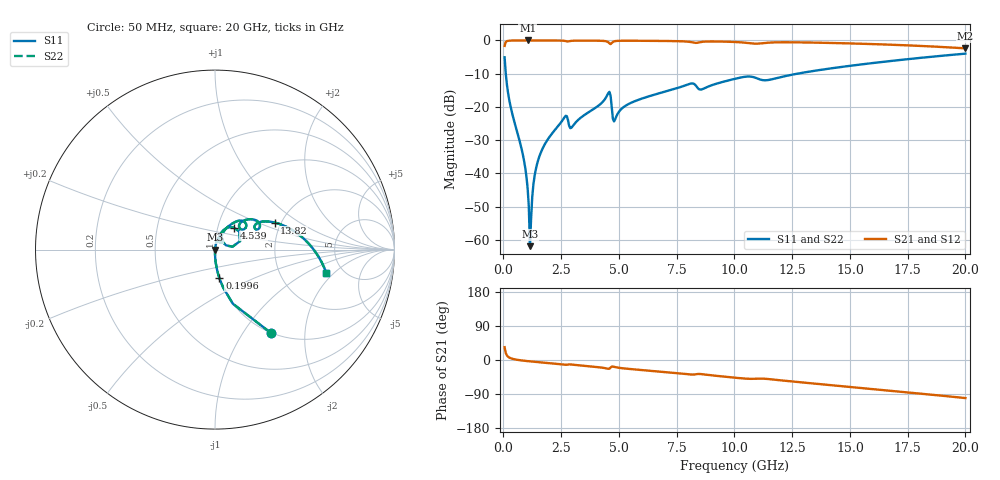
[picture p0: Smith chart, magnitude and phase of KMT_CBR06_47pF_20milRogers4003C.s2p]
! Data measured by Modelithics Inc. support@modelithics.com 813-866-6335
! KEMET CBR0603 47pF, Pad Width= 0.851mm, Pad Length= 0.64mm, Pad Gap= 0.62mm, 20mil Rogers 4003C substrate Data, January 2022
# hz S ma R 50
! 2 Port Network Data from SP1.SP block
! freq  magS11  angS11  magS21  angS21  magS12  angS12  magS22  angS22
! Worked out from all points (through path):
!   401 points, 50 MHz to 20 GHz, reference 50 ohm
!   highest |S21| = -0.01 dB at 1.048 GHz (marker M1); lowest = -2.4 dB at 20 GHz (marker M2)
!   group delay of S21, straight-line fit = 14 ps
!   lowest |S11| = -61.9 dB at 1.147 GHz (marker M3), VSWR 1.00, Z = 50.1 - j0.0562 ohm
!   |S11| at or under -10 dB: 100.6 MHz to 12.73 GHz (12.63 GHz wide, 197 % of centre)
!   |S22| runs from -61.9 to -4.0 dB; largest |S21 - S12| = 0
!   S11 on the Smith chart (normalised r, x): 50 MHz: 1.00, -1.34; 199.6 MHz: 1.00, -0.33; 4.539 GHz: 1.19, +0.30; 13.82 GHz: 1.85, +0.64; 20 GHz: 3.72, -1.60
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5e7  0.5586 -56.2  0.8291 33.8  0.8291 33.8  0.5586 -56.2
1.99625e8  0.1619 -81.2  0.9865 8.7  0.9865 8.7  0.1619 -81.2
8.48e8  0.01857 -90.0  0.9993 -1.6  0.9993 -1.6  0.01857 -90.0
9.97625e8  0.008804 -89.0  0.9994 -2.7  0.9994 -2.7  0.008804 -89.0
1.0475e9  0.005925 -87.4  0.9994 -3.0  0.9994 -3.0  0.005925 -87.4
1.14725e9  0.0008034 -44.3  0.9993 -3.6  0.9993 -3.6  0.0008034 -44.3
1.247e9  0.00447 77.6  0.9993 -4.2  0.9993 -4.2  0.00447 77.6
1.34675e9  0.009075 81.0  0.9992 -4.8  0.9992 -4.8  0.009075 81.0
1.4465e9  0.01345 81.7  0.9992 -5.4  0.9992 -5.4  0.01345 81.7
1.795625e9  0.02763 81.0  0.9987 -7.3  0.9987 -7.3  0.02763 81.0
2.6435e9  0.06992 67.9  0.9857 -12.3  0.9857 -12.3  0.06992 67.9
2.94275e9  0.0486 63.0  0.9862 -12.0  0.9862 -12.0  0.0486 63.0
3.391625e9  0.07074 72.8  0.9943 -14.8  0.9943 -14.8  0.07074 72.8
4.53875e9  0.1612 49.6  0.9401 -23.2  0.9401 -23.2  0.1612 49.6
4.838e9  0.06542 52.4  0.9768 -18.8  0.9768 -18.8  0.06542 52.4
5.386625e9  0.1091 64.7  0.99 -23.2  0.99 -23.2  0.1091 64.7
6.73325e9  0.16 58.5  0.9839 -30.4  0.9839 -30.4  0.16 58.5
1.0025e10  0.2648 39.8  0.9477 -46.7  0.9477 -46.7  0.2648 39.8
1.336662e10  0.345 26.8  0.9289 -61.7  0.9289 -61.7  0.345 26.8
1.38155e10  0.3644 24.5  0.9224 -64.2  0.9224 -64.2  0.3644 24.5
1.670825e10  0.4882 8.4  0.8643 -80.7  0.8643 -80.7  0.4882 8.4
2e10  0.633 -11.7  0.7597 -100.5  0.7597 -100.5  0.633 -11.7
